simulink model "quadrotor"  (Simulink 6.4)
settings: Solver=FixedStepDiscrete  SolverMode=SingleTasking  StartTime=0.0  StopTime=10.0  FixedStep=0.01  RelTol=1e-3
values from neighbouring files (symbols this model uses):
  v_batt = single(11.1)    [par.m]
undefined symbols (not defined in the file or in its folder): float, uint
libraries: simulink x5, aerosimlib x4, cstblocks x3

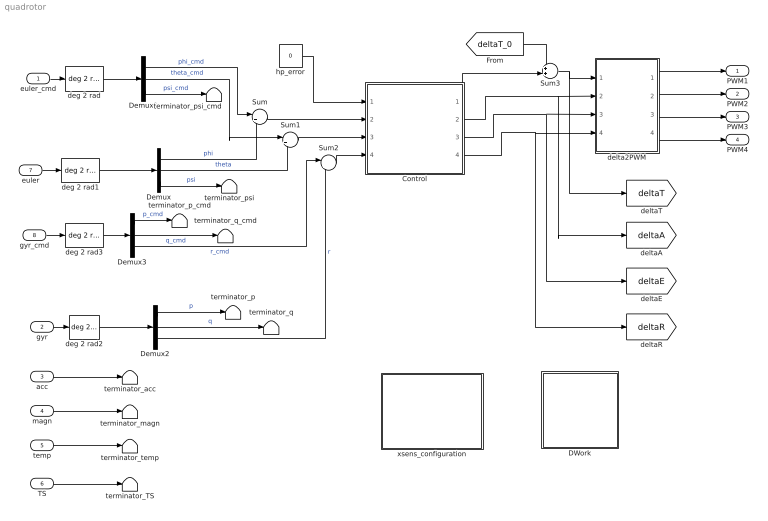
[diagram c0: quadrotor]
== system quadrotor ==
  euler_cmd : Inport  PortDimensions=3  DataType=single
  gyr : Inport  Port=2  PortDimensions=3  DataType=single
  acc : Inport  Port=3  PortDimensions=3  DataType=single
  magn : Inport  Port=4  PortDimensions=3  DataType=single
  temp : Inport  Port=5  PortDimensions=1  DataType=single
  TS : Inport  Port=6  PortDimensions=1  DataType=uint16
  euler : Inport  Port=7  PortDimensions=3  DataType=single
  gyr_cmd : Inport  Port=8  PortDimensions=3  DataType=single
  Control : Subsystem
  DWork : Subsystem
  Demux{,1..3} (4 alike) : Demux  Outputs=3
  Sum : Sum  Inputs=|+-
  Sum1 : Sum  Inputs=|+-
  Sum2 : Sum  Inputs=|+-
  Sum3 : Sum  Inputs=++|
  deg 2 rad{,1..3} (4 alike) : aerosimlib/Unit Conversion/Angular position/deg 2 rad  SystemSampleTime=-1
  delta2PWM : Subsystem
  hp_error : Constant  Value=0
  terminator_TS : Terminator
  terminator_acc : Terminator
  terminator_magn : Terminator
  terminator_p : Terminator
  terminator_p_cmd : Terminator
  terminator_psi : Terminator
  terminator_psi_cmd : Terminator
  terminator_q : Terminator
  terminator_q_cmd : Terminator
  terminator_temp : Terminator
  xsens_configuration : Subsystem
  PWM1 : Outport
  PWM2 : Outport  Port=2
  PWM3 : Outport  Port=3
  PWM4 : Outport  Port=4
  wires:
  delta2PWM/1(PWM1) -> PWM1/1
  delta2PWM/2(PWM2) -> PWM2/1
  delta2PWM/3(PWM3) -> PWM3/1
  delta2PWM/4(PWM4) -> PWM4/1
  acc/1 -> terminator_acc/1
  temp/1 -> terminator_temp/1
  TS/1 -> terminator_TS/1
  Demux/3 -> terminator_psi/1  "psi"
  Demux1/1 -> Sum/1  "phi_cmd"
  Demux1/2 -> Sum1/1  "theta_cmd"
  Demux1/3 -> terminator_psi_cmd/1  "psi_cmd"
  Control/2(deltaA) -> delta2PWM/2(deltaA), [deltaA]
  Control/3(deltaE) -> delta2PWM/3(deltaE), [deltaE]
  Sum/1 -> Control/2(phi_error)
  Sum1/1 -> Control/3(theta_error)
  euler_cmd/1 -> deg 2 rad/1
  deg 2 rad/1 -> Demux1/1
  euler/1 -> deg 2 rad1/1
  deg 2 rad1/1 -> Demux/1
  gyr/1 -> deg 2 rad2/1
  Demux2/1 -> terminator_p/1  "p"
  Demux2/2 -> terminator_q/1  "q"
  Demux2/3 -> Sum2/2  "r"
  Demux3/3 -> Sum2/1  "r_cmd"
  Sum2/1 -> Control/4(r_error)
  hp_error/1 -> Control/1(hp_error)
  deg 2 rad2/1 -> Demux2/1
  Demux/1 -> Sum/2  "phi"
  Demux/2 -> Sum1/2  "theta"
  gyr_cmd/1 -> deg 2 rad3/1
  deg 2 rad3/1 -> Demux3/1
  Demux3/2 -> terminator_q_cmd/1  "q_cmd"
  Demux3/1 -> terminator_p_cmd/1  "p_cmd"
  Sum3/1 -> delta2PWM/1(deltaT), [deltaT]
  [deltaT_0] -> Sum3/1
  Control/1(deltaT) -> Sum3/2
  magn/1 -> terminator_magn/1
  Control/4(deltaR) -> delta2PWM/4(deltaR), [deltaR]

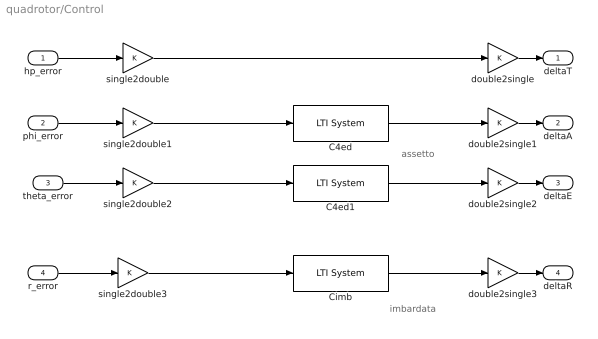
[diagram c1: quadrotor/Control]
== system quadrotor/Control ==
  note: assetto
  note: imbardata
  hp_error : Inport
  phi_error : Inport  Port=2
  theta_error : Inport  Port=3
  r_error : Inport  Port=4
  C4ed : cstblocks/LTI System  SystemSampleTime=-1  sys=assetto  IC=[]
  C4ed1 : cstblocks/LTI System  SystemSampleTime=-1  sys=assetto  IC=[]
  Cimb : cstblocks/LTI System  SystemSampleTime=-1  sys=imba  IC=[]
  double2single{,1..3} (4 alike) : Gain  OutDataTypeMode=Specify via dialog  OutDataType=float('single')
  single2double{,1..3} (4 alike) : Gain  OutDataTypeMode=Specify via dialog  OutDataType=float('double')
  deltaT : Outport
  deltaA : Outport  Port=2
  deltaE : Outport  Port=3
  deltaR : Outport  Port=4
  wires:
  hp_error/1 -> single2double/1
  phi_error/1 -> single2double1/1
  C4ed/1 -> double2single1/1
  theta_error/1 -> single2double2/1
  C4ed1/1 -> double2single2/1
  Cimb/1 -> double2single3/1
  r_error/1 -> single2double3/1
  single2double1/1 -> C4ed/1
  single2double2/1 -> C4ed1/1
  single2double3/1 -> Cimb/1
  double2single/1 -> deltaT/1
  double2single1/1 -> deltaA/1
  double2single2/1 -> deltaE/1
  double2single3/1 -> deltaR/1
  single2double/1 -> double2single/1

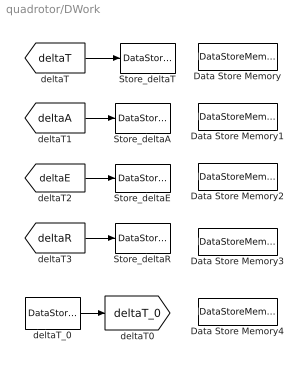
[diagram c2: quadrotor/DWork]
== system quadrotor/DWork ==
  Data Store Memory : DataStoreMemory  DataStoreName=DELTA_T  ReadBeforeWriteMsg=warning  WriteAfterWriteMsg=warning  WriteAfterReadMsg=warning  InitialValue=0  DataType=single
  Data Store Memory1 : DataStoreMemory  DataStoreName=DELTA_A  ReadBeforeWriteMsg=warning  WriteAfterWriteMsg=warning  WriteAfterReadMsg=warning  InitialValue=0  DataType=single
  Data Store Memory2 : DataStoreMemory  DataStoreName=DELTA_E  ReadBeforeWriteMsg=warning  WriteAfterWriteMsg=warning  WriteAfterReadMsg=warning  InitialValue=0  DataType=single
  Data Store Memory3 : DataStoreMemory  DataStoreName=DELTA_R  ReadBeforeWriteMsg=warning  WriteAfterWriteMsg=warning  WriteAfterReadMsg=warning  InitialValue=0  DataType=single
  Data Store Memory4 : DataStoreMemory  DataStoreName=DELTA_T_0  ReadBeforeWriteMsg=warning  WriteAfterWriteMsg=warning  WriteAfterReadMsg=warning  InitialValue=0  DataType=single
  Store_deltaA : DataStoreWrite  DataStoreName=DELTA_A  SampleTime=-1
  Store_deltaE : DataStoreWrite  DataStoreName=DELTA_E  SampleTime=-1
  Store_deltaR : DataStoreWrite  DataStoreName=DELTA_R  SampleTime=-1
  Store_deltaT : DataStoreWrite  DataStoreName=DELTA_T  SampleTime=-1
  deltaT_0 : DataStoreRead  DataStoreName=DELTA_T_0  SampleTime=-1
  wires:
  [deltaT] -> Store_deltaT/1
  [deltaA] -> Store_deltaA/1
  [deltaE] -> Store_deltaE/1
  [deltaR] -> Store_deltaR/1
  deltaT_0/1 -> [deltaT_0]

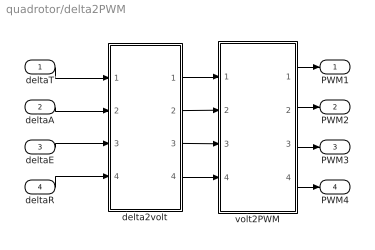
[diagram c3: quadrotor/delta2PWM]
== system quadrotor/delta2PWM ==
  deltaT : Inport
  deltaA : Inport  Port=2
  deltaE : Inport  Port=3
  deltaR : Inport  Port=4
  delta2volt : Subsystem
  volt2PWM : Subsystem
  PWM1 : Outport
  PWM2 : Outport  Port=2
  PWM3 : Outport  Port=3
  PWM4 : Outport  Port=4
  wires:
  delta2volt/1(V1) -> volt2PWM/1(V1)
  delta2volt/2(V2) -> volt2PWM/2(V2)
  delta2volt/3(V3) -> volt2PWM/3(V3)
  delta2volt/4(V4) -> volt2PWM/4(V4)
  volt2PWM/1(PWM1) -> PWM1/1
  volt2PWM/2(PWM2) -> PWM2/1
  volt2PWM/3(PWM3) -> PWM3/1
  volt2PWM/4(PWM4) -> PWM4/1
  deltaT/1 -> delta2volt/1(deltaT)
  deltaA/1 -> delta2volt/2(deltaA)
  deltaE/1 -> delta2volt/3(deltaE)
  deltaR/1 -> delta2volt/4(deltaR)

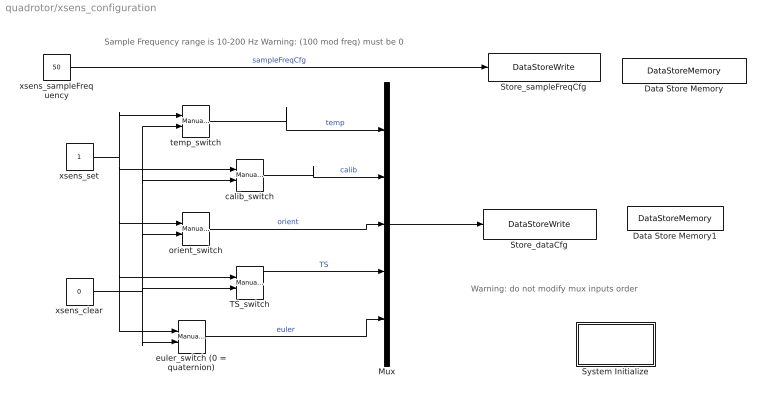
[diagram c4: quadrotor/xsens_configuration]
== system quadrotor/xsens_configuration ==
  note: Warning: do not modify mux inputs order
  note: Sample Frequency range is 10-200 Hz Warning: (100 mod freq) must be 0
  Data Store Memory : DataStoreMemory  DataStoreName=xsensSampleFreqCfg  ReadBeforeWriteMsg=warning  WriteAfterWriteMsg=warning  WriteAfterReadMsg=warning  InitialValue=0  DataType=uint16
  Data Store Memory1 : DataStoreMemory  DataStoreName=xsensDataCfg  ReadBeforeWriteMsg=warning  WriteAfterWriteMsg=warning  WriteAfterReadMsg=warning  InitialValue=[0 0 0 0 0]  DataType=uint8  OutDataType=ciccio
  Mux : Mux  Inputs=5
  Store_dataCfg : DataStoreWrite  DataStoreName=xsensDataCfg  SampleTime=-1
  Store_sampleFreqCfg : DataStoreWrite  DataStoreName=xsensSampleFreqCfg  SampleTime=-1
  System Initialize : Subsystem  mask(System Initialize){ShowInLibBrowser=0}
      mask prompts: ShowInLibBrowser "Mask Parameter 1:"
      mask help: Add code to a systems Initialize function
  TS_switch : simulink/Signal Routing/Manual Switch  SystemSampleTime=-1  sw=1  action=0
  calib_switch : simulink/Signal Routing/Manual Switch  SystemSampleTime=-1  sw=1  action=0
  euler_switch (0 = quaternion) : simulink/Signal Routing/Manual Switch  SystemSampleTime=-1  sw=1  action=0
  orient_switch : simulink/Signal Routing/Manual Switch  SystemSampleTime=-1  sw=1  action=0
  temp_switch : simulink/Signal Routing/Manual Switch  SystemSampleTime=-1  sw=0  action=0
  xsens_clear : Constant  Value=0  OutDataTypeMode=uint8
  xsens_sampleFrequency : Constant  Value=50  OutDataTypeMode=uint16
  xsens_set : Constant  OutDataTypeMode=uint8
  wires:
  xsens_clear/1 -> TS_switch/2, temp_switch/2, calib_switch/2, orient_switch/2, euler_switch (0 = quaternion)/2
  xsens_set/1 -> temp_switch/1, calib_switch/1, orient_switch/1, TS_switch/1, euler_switch (0 = quaternion)/1
  Mux/1 -> Store_dataCfg/1
  temp_switch/1 -> Mux/1  "temp"
  calib_switch/1 -> Mux/2  "calib"
  orient_switch/1 -> Mux/3  "orient"
  TS_switch/1 -> Mux/4  "TS"
  euler_switch (0 = quaternion)/1 -> Mux/5  "euler"
  xsens_sampleFrequency/1 -> Store_sampleFreqCfg/1  "sampleFreqCfg"

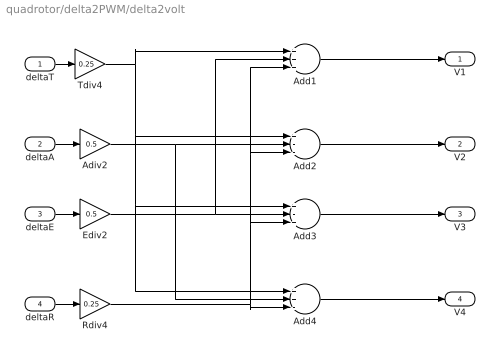
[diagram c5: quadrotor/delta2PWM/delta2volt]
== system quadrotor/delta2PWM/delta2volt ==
  deltaT : Inport
  deltaA : Inport  Port=2
  deltaE : Inport  Port=3
  deltaR : Inport  Port=4
  Add1 : Sum  Inputs=+++  OutScaling=2^-10
  Add2 : Sum  Inputs=+--  OutScaling=2^-10
  Add3 : Sum  Inputs=+-+  OutScaling=2^-10
  Add4 : Sum  Inputs=++-  OutScaling=2^-10
  Adiv2 : Gain  Gain=0.5
  Ediv2 : Gain  Gain=0.5
  Rdiv4 : Gain  Gain=0.25
  Tdiv4 : Gain  Gain=0.25
  V1 : Outport
  V2 : Outport  Port=2
  V3 : Outport  Port=3
  V4 : Outport  Port=4
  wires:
  deltaE/1 -> Ediv2/1
  deltaT/1 -> Tdiv4/1
  deltaA/1 -> Adiv2/1
  deltaR/1 -> Rdiv4/1
  Add4/1 -> V4/1
  Add3/1 -> V3/1
  Add2/1 -> V2/1
  Add1/1 -> V1/1
  Rdiv4/1 -> Add4/3, Add3/3, Add1/3, Add2/3
  Adiv2/1 -> Add2/2, Add4/2
  Ediv2/1 -> Add1/2, Add3/2
  Tdiv4/1 -> Add1/1, Add2/1, Add4/1, Add3/1

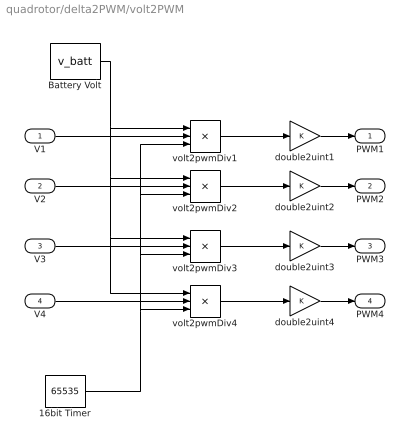
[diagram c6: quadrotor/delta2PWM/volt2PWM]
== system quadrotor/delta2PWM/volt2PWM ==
  V1 : Inport
  V2 : Inport  Port=2
  V3 : Inport  Port=3
  V4 : Inport  Port=4
  16bit Timer : Constant  Value=65535  OutDataTypeMode=uint16
  Battery Volt : Constant  Value=v_batt  OutDataTypeMode=single
  double2uint{1..4} (4 alike) : Gain  OutDataTypeMode=Specify via dialog  OutDataType=uint(16)
  volt2pwmDiv{1..4} (4 alike) : Product  Inputs=/**  OutScaling=2^-10
  PWM1 : Outport
  PWM2 : Outport  Port=2
  PWM3 : Outport  Port=3
  PWM4 : Outport  Port=4
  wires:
  V1/1 -> volt2pwmDiv1/2
  volt2pwmDiv1/1 -> double2uint1/1
  Battery Volt/1 -> volt2pwmDiv1/1, volt2pwmDiv3/1, volt2pwmDiv4/1, volt2pwmDiv2/1
  16bit Timer/1 -> volt2pwmDiv1/3, volt2pwmDiv2/3, volt2pwmDiv3/3, volt2pwmDiv4/3
  V2/1 -> volt2pwmDiv2/2
  V3/1 -> volt2pwmDiv3/2
  V4/1 -> volt2pwmDiv4/2
  volt2pwmDiv2/1 -> double2uint2/1
  volt2pwmDiv3/1 -> double2uint3/1
  volt2pwmDiv4/1 -> double2uint4/1
  double2uint1/1 -> PWM1/1
  double2uint2/1 -> PWM2/1
  double2uint3/1 -> PWM3/1
  double2uint4/1 -> PWM4/1

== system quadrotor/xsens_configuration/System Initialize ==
